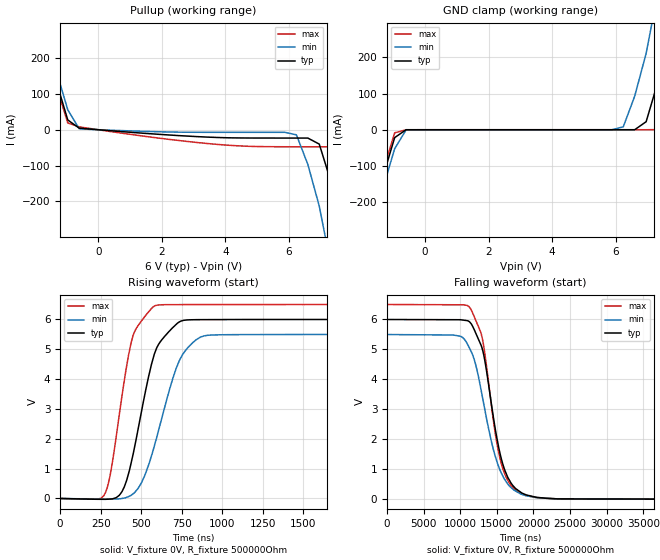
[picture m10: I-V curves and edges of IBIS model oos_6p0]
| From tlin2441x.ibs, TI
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|   oos_6p0 Model
[Model]   oos_6p0
Model_type   Open_source
Polarity   Non-Inverting
Vmeas = 3
Vref = 0
Cref = 2pF
Rref = 500000
|   typ   min   max
C_comp   1.386pF   1.379pF   1.431pF
|  Where Nom  PVT is Nominal Process, 6.0V,   27C
|   Fast PVT is Strong Process,  6.5,   -40C
|   Slow PVT is Weak Process,   5.5V,   150C
[Voltage Range]   6   5.5   6.5
|Junction Temperature
[Temperature Range]   27   150   -40
[Pullup Reference]   6   5.5   6.5
[Pulldown Reference]   0   0   0
[Power Clamp Reference]   6   5.5   6.5
[GND Clamp Reference]   0   0   0
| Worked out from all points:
|   slope of the pullup table from 0 to 0.9 V, typ, clamps not added: 142 ohm
|   GND clamp passes 1 mA (typ) near -0.62 V on its own axis
|   falling waveform, V_fixture 0V, R_fixture 500000Ohm: 20-80 % time 2.56us typ, 3.03us min, 2.35us max; typ from 6 V to 0 V
|   rising waveform, V_fixture 0V, R_fixture 500000Ohm: 20-80 % time 141ns typ, 175ns min, 112ns max; typ from 0 V to 6 V
[GND Clamp]
|   Voltage   I(typ)   I(min)   I(max)
-6V       -2.668A    -2.648A    -2.692A
-1.68V    -289.1mA   -303.9mA   -286mA
-1.32V    -127.6mA   -159.7mA   -112.6mA
-960mV    -21.88mA   -52.63mA   -8.634mA
-600mV    -4.543uA   -605.5uA   -3.864uA
6.24V     755.2pA    8.034mA    665.6pA
6.96V     22.18mA    211.1mA    27.73nA
7.32V     128.9mA    375.3mA    381.8uA
7.68V     290.7mA    563.1mA    66.39mA
8.076V    500.6mA    775.5mA    233.4mA
8.4V      675.9mA    951mA      405.1mA
12V       2.662A     2.932A     2.393A
[Pullup]
|   Voltage   I(typ)   I(min)   I(max)
-6V       2.668A     2.658A     2.683A
-1.68V    294.9mA    308.2mA    294.8mA
-1.32V    134mA      163.9mA    122.7mA
-960mV    27.31mA    55.77mA    18.92mA
-600mV    4.456mA    2.646mA    8.085mA
6.24V     -23.26mA   -14.23mA   -47.62mA
6.96V     -40.14mA   -213.4mA   -47.67mA
7.32V     -142.9mA   -376.5mA   -47.89mA
7.68V     -300.5mA   -563.7mA   -99.16mA
8.04V     -489.9mA   -756.1mA   -236.9mA
8.4V      -684.1mA   -950.6mA   -425.6mA
12V       -2.678A    -2.927A    -2.427A
[Ramp]
R_load = 500000
|   typ   min   max
dV/dt_r   3.59899/1.40627e-07   3.29794/1.7468e-07   3.89939/1.12081e-07
dV/dt_f   3.59899/2.5589e-06   3.29794/3.02819e-06   3.89939/2.35088e-06
[Falling Waveform]
V_fixture = 0V
V_fixture_min = 0V
V_fixture_max = 0V
R_fixture = 500000Ohm
C_fixture = 0F
|   Time   V(typ)   V(min)   V(max)
0s        5.998V     5.497V     6.499V
10.03us   5.991V     5.44V      6.489V
11.43us   5.875V     4.963V     6.351V
12.15us   5.526V     4.452V     5.954V
13.01us   5.018V     3.438V     5.373V
14.81us   2.306V     1.412V     2.152V
15.55us   1.413V     907.5mV    1.248V
16.66us   658.4mV    459.6mV    556.8mV
18.26us   236.4mV    180.3mV    196.1mV
50us      38.35uV    223.2uV    30.89uV
[Rising Waveform]
V_fixture = 0V
V_fixture_min = 0V
V_fixture_max = 0V
R_fixture = 500000Ohm
C_fixture = 0F
|   Time   V(typ)   V(min)   V(max)
0s        38.35uV    223.2uV    30.89uV
268.3ns   -27.89mV   -22.66mV   88.58mV
308.4ns   -19.12mV   -20.37mV   786.4mV
380.3ns   221.7mV    -725uV     3.404V
460.3ns   1.761V     206.9mV    5.606V
562.9ns   4.492V     1.428V     6.363V
632.4ns   5.355V     2.81V      6.491V
771.6ns   5.975V     4.952V     6.496V
1.016us   5.994V     5.486V     6.498V
50us      5.998V     5.497V     6.499V
